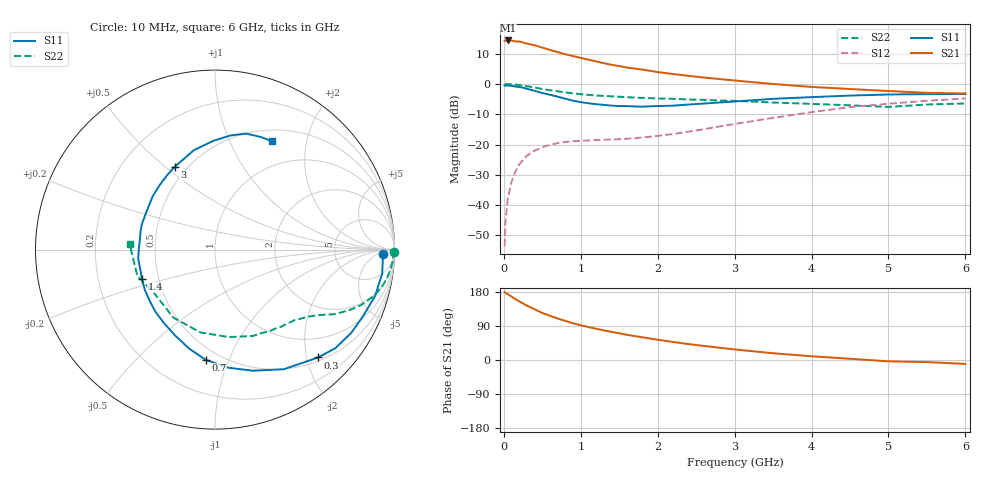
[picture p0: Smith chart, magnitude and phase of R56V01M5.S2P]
! SIEMENS Small Signal Semiconductors
! BFR183
! Si NPN RF Bipolar Junction Transistor in SOT23
! VCE = 6 V  IC = 1.5 mA
! Common Emitter S-Parameters:  May  1996
# GHz  S  MA  R  50
!  f  S11  S21  S12  S22
! GHz  MAG  ANG  MAG  ANG  MAG  ANG  MAG  ANG
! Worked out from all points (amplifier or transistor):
!   36 points, 10 MHz to 6 GHz, reference 50 ohm
!   highest |S21| = 14.3 dB at 50 MHz (marker M1)
!   |S21| within 3 dB of that: start of sweep to 582.7 MHz
!   unconditionally stable (mu >= 1): 1.529 GHz to 2.888 GHz
!   at 250 MHz: K = 0.19, MSG = 19.3 dB, |S12| = -25.0 dB
!   at 1.4 GHz: K = 0.94, MSG = 12.3 dB, |S12| = -18.4 dB
!   at 6 GHz: K = 0.92, MSG = 0.8 dB, |S12| = -4.8 dB
!   S11 on the Smith chart (normalised r, x): 10 MHz: 27, -12; 300 MHz: 0.57, -2.22; 700 MHz: 0.42, -0.83; 1.4 GHz: 0.40, -0.16; 3 GHz: 0.43, +0.54; 6 GHz: 0.64, +1.45
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0.01  0.9389 -1.6  5.168 179.1  0.0021 93.2  0.9973 -0.7
0.02  0.9364 -3.1  5.085 177.4  0.0051 86.3  0.9897 -1.1
0.05  0.9411 -8.1  5.215 173.8  0.0125 84.2  0.9947 -3.1
0.1  0.9287 -16.1  5.2 167.6  0.0242 80.8  0.9842 -6.2
0.15  0.9052 -23.9  5.033 160.7  0.0357 75.8  0.9733 -9.1
0.2  0.8897 -31.4  5.006 154.8  0.0465 72.1  0.9572 -11.8
0.25  0.8668 -39.3  4.826 149.0  0.0561 67.5  0.937 -14.5
0.3  0.8315 -46.3  4.626 143.5  0.0652 64.3  0.9164 -16.7
0.4  0.769 -60.1  4.352 133.8  0.0794 57.8  0.8712 -20.7
0.5  0.7071 -72.6  3.976 124.2  0.09 52.3  0.825 -24.0
0.6  0.6618 -83.7  3.635 116.6  0.0988 48.0  0.7861 -26.4
0.7  0.6163 -94.8  3.352 109.6  0.1054 44.6  0.7561 -28.4
0.9  0.5286 -114.6  2.882 96.9  0.1133 40.3  0.6985 -31.4
1.1  0.4797 -133.8  2.513 87.0  0.1166 38.5  0.6585 -34.1
1.4  0.4388 -158.2  2.067 74.2  0.1205 38.9  0.6236 -37.6
1.8  0.4219 172.6  1.72 59.9  0.1308 44.6  0.5884 -42.5
2.2  0.4376 149.9  1.455 47.6  0.1486 50.4  0.5682 -48.9
3  0.5126 116.1  1.138 27.9  0.2181 55.6  0.5258 -66.2
3.5  0.5669 101.9  0.997 17.8  0.2752 53.3  0.4931 -81.2
4.5  0.6418 82.3  0.824 3.3  0.4139 41.6  0.4442 -121.5
5.5  0.6777 67.7  0.713 -5.5  0.5278 26.2  0.457 -161.2
6  0.6812 62.4  0.695 -10.3  0.5747 16.5  0.4757 176.5
